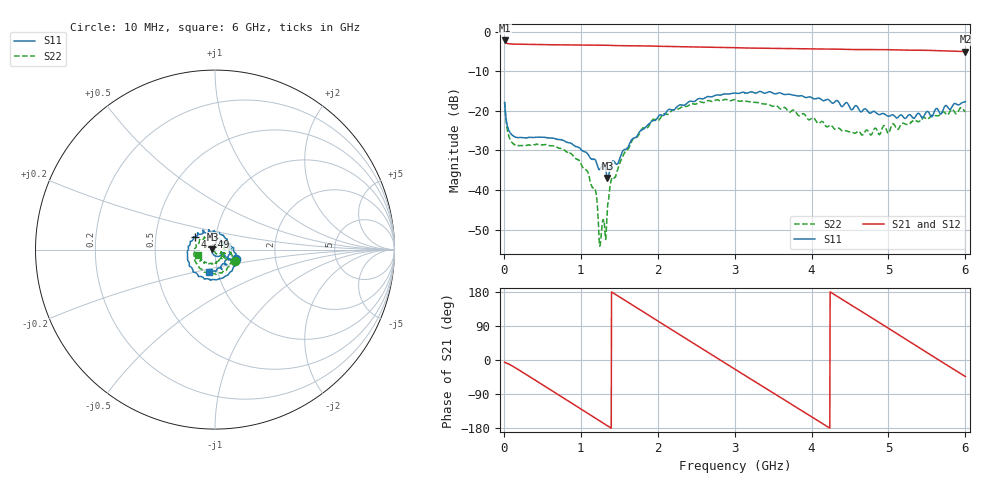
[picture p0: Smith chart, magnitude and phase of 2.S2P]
!Agilent Technologies,E5071C,MY46316741,A.11.02
!Date: Thu Jul 30 16:11:41 2020
!Data & Calibration Information:
!Freq	S11:SOLT4(ON)	S21:SOLT4(ON)	S12:SOLT4(ON)	S22:SOLT4(ON)
!PortZ  Port1:50+j0  Port2:50+j0
!Above PortZ is port z conversion or system Z0 setting when saving the data.
!When reading, reference impedance value at option line is always used.
# Hz S dB R 50
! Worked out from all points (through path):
!   1561 points, 10 MHz to 6 GHz, reference 50 ohm
!   highest |S21| = -2.18 dB at 10 MHz (marker M1); lowest = -5.0 dB at 6 GHz (marker M2)
!   group delay of S21, straight-line fit = 352 ps
!   lowest |S11| = -36.9 dB at 1.346 GHz (marker M3), VSWR 1.03, Z = 48.6 + j0.231 ohm
!   |S11| at or under -10 dB: start of sweep to end of sweep
!   |S22| runs from -54.2 to -17.1 dB; largest |S21 - S12| = 0.0091
!   S11 on the Smith chart (normalised r, x): 10 MHz: 1.25, -0.14; 4.249 GHz: 0.79, +0.11; 6 GHz: 0.91, -0.24
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1e7  -17.84 -25.1  -2.18 -5.4  -2.18 -5.5  -17.75 -28.3
6.375641e7  -24.87 -29.2  -3.02 -10.5  -3.01 -10.5  -26.34 -35.6
1.290321e8  -26.42 -22.5  -3.11 -18.1  -3.11 -18.1  -28.34 -25.3
5.898013e8  -26.82 -45.8  -3.26 -76.5  -3.25 -76.6  -28.77 -37.6
1.012173e9  -29.90 -98.0  -3.34 -130.5  -3.34 -130.7  -33.80 -77.4
1.184962e9  -32.31 -131.0  -3.38 -152.6  -3.38 -152.8  -39.67 -102.4
1.250237e9  -34.70 -160.6  -3.39 -161.0  -3.38 -161.2  -53.98 -162.7
1.346231e9  -36.94 170.4  -3.39 -173.4  -3.39 -173.6  -44.94 63.4
1.396147e9  -33.18 141.1  -3.43 -180.0  -3.42 179.8  -37.51 83.0
1.553577e9  -29.98 98.6  -3.51 160.1  -3.50 159.9  -31.13 59.6
1.799321e9  -24.75 51.9  -3.55 128.9  -3.55 128.6  -24.48 27.7
2.006667e9  -21.42 23.2  -3.65 102.2  -3.64 102.0  -22.40 2.6
2.267769e9  -18.67 -10.2  -3.75 69.0  -3.74 68.6  -19.51 -28.4
2.567269e9  -16.92 -41.5  -3.86 31.1  -3.85 30.7  -17.77 -62.9
3.005e9  -15.48 -87.4  -4.01 -24.4  -4.00 -24.9  -17.12 -115.5
3.504167e9  -15.57 -138.4  -4.19 -87.3  -4.18 -87.8  -18.79 -177.8
4.007173e9  -16.71 171.8  -4.33 -150.7  -4.31 -151.3  -21.79 112.3
4.249077e9  -17.68 147.9  -4.37 178.8  -4.35 178.1  -23.60 73.9
4.671449e9  -19.77 93.6  -4.48 125.5  -4.48 124.8  -25.97 -0.5
5.001667e9  -21.34 47.1  -4.51 83.3  -4.51 82.5  -25.68 -45.3
5.520032e9  -20.27 -34.3  -4.69 17.2  -4.68 16.4  -21.93 -106.4
6e9  -17.66 -103.7  -4.99 -43.6  -4.97 -44.5  -20.21 -162.2
